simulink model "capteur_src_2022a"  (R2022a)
settings: Solver=VariableStepAuto  StartTime=0.0  StopTime=10.0  RelTol=1e-3
libraries: simulink x1

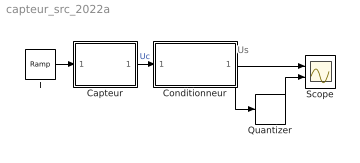
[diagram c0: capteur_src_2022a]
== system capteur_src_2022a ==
  note: Us
  Capteur : Subsystem
  Conditionneur : Subsystem
  Quantizer : Quantizer  QuantizationInterval=5/1024
  Scope : Scope  NumInputPorts=2
  T : simulink/Sources/Ramp  slope=13  start=0  InitialOutput=70
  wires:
  T/1 -> Capteur/1(T)
  Capteur/1(Uc) -> Conditionneur/1(In1)  "Uc"
  Conditionneur/1(Out1) -> Quantizer/1, Scope/1
  Quantizer/1 -> Scope/2

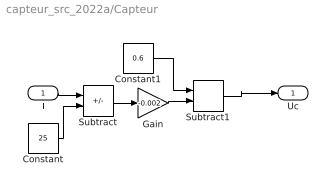
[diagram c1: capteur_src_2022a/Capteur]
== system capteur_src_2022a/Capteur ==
  T : Inport
  Constant : Constant  Value=25
  Constant1 : Constant  Value=0.6
  Gain : Gain  Gain=-0.002
  Subtract : Sum  Inputs=+-
  Subtract1 : Sum
  Uc : Outport
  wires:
  T/1 -> Subtract/1
  Constant/1 -> Subtract/2
  Subtract/1 -> Gain/1
  Gain/1 -> Subtract1/2
  Constant1/1 -> Subtract1/1
  Subtract1/1 -> Uc/1

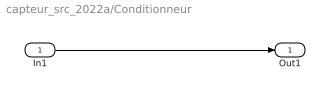
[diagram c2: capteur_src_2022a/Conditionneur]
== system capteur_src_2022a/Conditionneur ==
  In1 : Inport
  Out1 : Outport
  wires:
  In1/1 -> Out1/1
